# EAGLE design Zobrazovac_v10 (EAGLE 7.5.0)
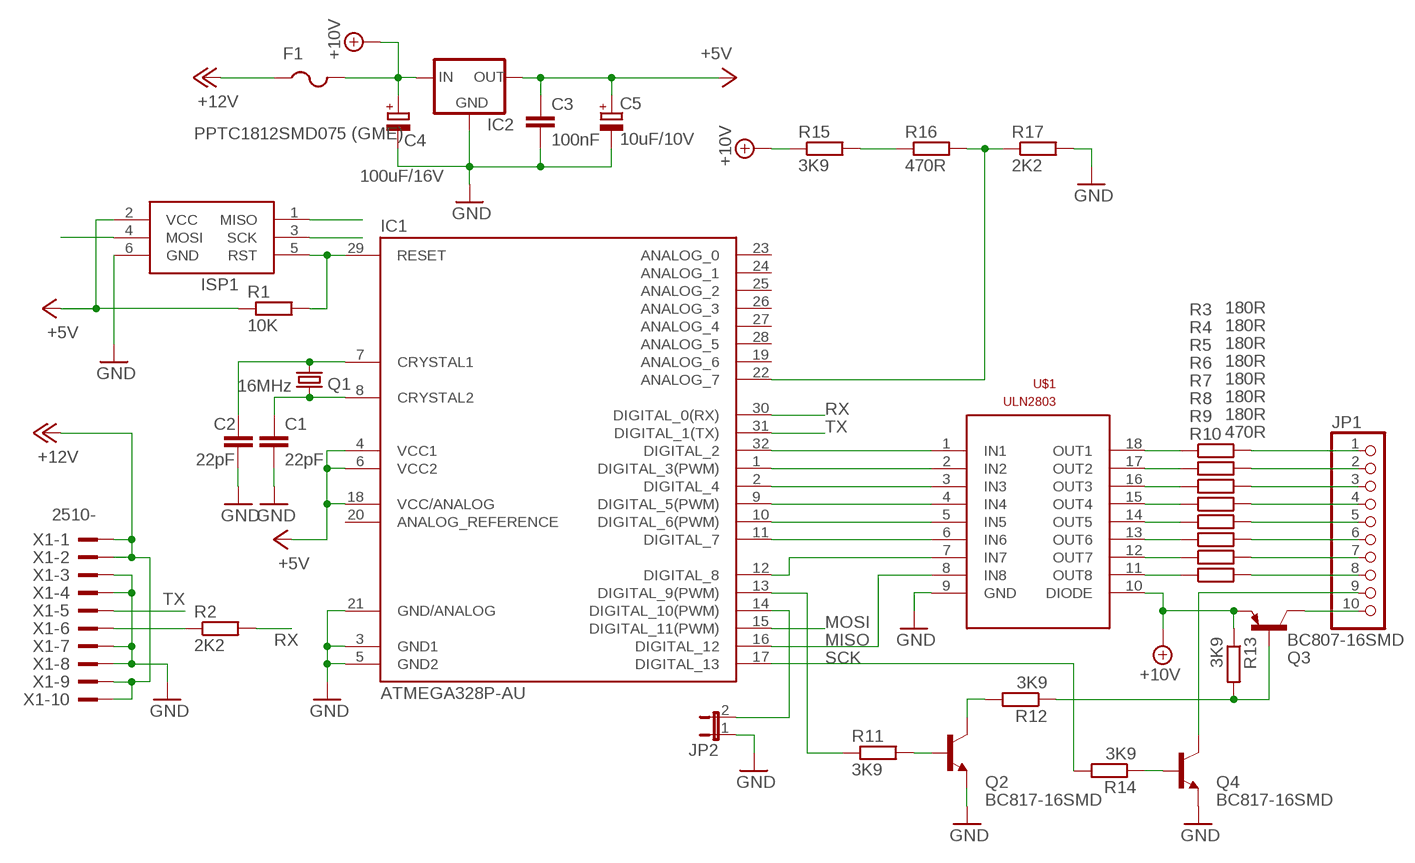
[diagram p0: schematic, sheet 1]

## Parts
C1  22pF  C-EUC1206  [C1206]
C2  22pF  C-EUC1206  [C1206]
C3  100nF  C-EUC1206  [C1206]
C4  100uF/16V  CPOL-EUSMCD  [SMC_D]
C5  10uF/10V  CPOL-EUSMCB  [SMC_B]
F1  PPTC1812SMD075 (GME)  PTCFUSE-1812  [1812]
IC1  ATMEGA328P-AU  ATMEGA168-AU  [TQFP32-08]
IC2  78LXX-SOT89  [SOT89]
ISP1  AVRISP-6  [AVRISP]
JP1  PINHD-1X10  [1X10]
JP2  JP1E  [JP1]
Q1  16MHz  CRYSTALSM49  [SM49]
Q2  BC817-16SMD  [SOT23-BEC]
Q3  BC807-16SMD  [SOT23-BEC]
Q4  BC817-16SMD  [SOT23-BEC]
R1  10K  R-EU_R1206  [R1206]
R2  2K2  R-EU_R1206  [R1206]
R3  180R  R-EU_R1206  [R1206]
R4  180R  R-EU_R1206  [R1206]
R5  180R  R-EU_R1206  [R1206]
R6  180R  R-EU_R1206  [R1206]
R7  180R  R-EU_R1206  [R1206]
R8  180R  R-EU_R1206  [R1206]
R9  180R  R-EU_R1206  [R1206]
R10  470R  R-EU_R1206  [R1206]
R11  3K9  R-EU_R1206  [R1206]
R12  3K9  R-EU_R1206  [R1206]
R13  3K9  R-EU_R1206  [R1206]
R14  3K9  R-EU_R1206  [R1206]
R15  3K9  R-EU_R1206  [R1206]
R16  470R  R-EU_R1206  [R1206]
R17  2K2  R-EU_R1206  [R1206]
U$1  ULN2803  [SO18L]
X1  2510-  [PAK100/2500-10]

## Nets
+5V: C3.1 C5.+ IC1.4(VCC1) IC1.6(VCC2) IC1.18(VCC/ANALOG) IC2.1(OUT) ISP1.2(VCC) R1.1
+10V [10V]: C4.+ F1.2 IC2.3(IN) Q3.E R13.1 R15.1 U$1.10(DIODE)
+12V [10V]: F1.1 X1.1 X1.2 X1.9 X1.10
GND [GND]: C1.2 C2.2 C3.2 C4.- C5.- IC1.3(GND1) IC1.5(GND2) IC1.21(GND/ANALOG) IC2.2(GND) ISP1.6(GND) JP2.1 Q2.E Q4.E R17.2 U$1.9(GND) X1.3 X1.4 X1.7 X1.8
MISO: IC1.16(DIGITAL_12) ISP1.1(MISO) U$1.8(IN8)
MOSI: IC1.15(DIGITAL_11(PWM)) ISP1.4(MOSI)
N$1 [OUT]: R3.1 U$1.18(OUT1)
N$2: R2.1 X1.6
N$3: C2.1 IC1.7(CRYSTAL1) Q1.2
N$4: C1.1 IC1.8(CRYSTAL2) Q1.1
N$5: JP1.1 R3.2
N$6: IC1.32(DIGITAL_2) U$1.1(IN1)
N$7: IC1.1(DIGITAL_3(PWM)) U$1.2(IN2)
N$8: IC1.2(DIGITAL_4) U$1.3(IN3)
N$9: IC1.9(DIGITAL_5(PWM)) U$1.4(IN4)
N$10: IC1.10(DIGITAL_6(PWM)) U$1.5(IN5)
N$11: IC1.11(DIGITAL_7) U$1.6(IN6)
N$12: IC1.12(DIGITAL_8) U$1.7(IN7)
N$13: IC1.14(DIGITAL_10(PWM)) JP2.2
N$14 [OUT]: R4.1 U$1.17(OUT2)
N$15 [OUT]: R5.1 U$1.16(OUT3)
N$16 [OUT]: R6.1 U$1.15(OUT4)
N$17 [OUT]: R7.1 U$1.14(OUT5)
N$18 [OUT]: R8.1 U$1.13(OUT6)
N$19 [OUT]: R9.1 U$1.12(OUT7)
N$20 [OUT]: R10.1 U$1.11(OUT8)
N$21: JP1.2 R4.2
N$22: JP1.3 R5.2
N$23: JP1.4 R6.2
N$24: JP1.5 R7.2
N$25: JP1.6 R8.2
N$26: JP1.7 R9.2
N$27 [10V]: JP1.8 R10.2
N$28: IC1.13(DIGITAL_9(PWM)) R11.1
N$29: Q2.B R11.2
N$30 [10V]: JP1.10 Q3.C
N$31: Q2.C R12.2
N$32: Q3.B R12.1 R13.2
N$33 [10V]: JP1.9 Q4.C
N$34: Q4.B R14.1
N$35: R15.2 R16.1
N$36: IC1.22(ANALOG_7) R16.2 R17.1
RST: IC1.29(RESET) ISP1.5(RST) R1.2
RX: IC1.30(DIGITAL_0(RX)) R2.2
SCK: IC1.17(DIGITAL_13) ISP1.3(SCK) R14.2
TX: IC1.31(DIGITAL_1(TX)) X1.5
Unconnected: IC1.19(ANALOG_6) IC1.20(ANALOG_REFERENCE) IC1.23(ANALOG_0) IC1.24(ANALOG_1) IC1.25(ANALOG_2) IC1.26(ANALOG_3) IC1.27(ANALOG_4) IC1.28(ANALOG_5)

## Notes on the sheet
- RX
- TX
- TX
- MOSI
- RX | MISO
- SCK

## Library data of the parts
C1-C3 = rcl:C-EU: CAPACITOR, European symbol
C4 C5 = rcl:CPOL-EU: POLARIZED CAPACITOR, European symbol
F1 = adafruit:PTCFUSE: PTC fuses, resettable thermistors
IC1 = Arduino-AVR:ATMEGA168
IC2 = v-reg-3:78LXX: VOLTAGE REGULATOR
ISP1 = adafruit:AVRISP: AVR ISP HEADER Standard 6 pin header for AVR programming
JP1 = pinhead:PINHD-1X10: PIN HEADER
JP2 = jumper:JP1E: JUMPER
Q1 = crystal:CRYSTAL: CRYSTAL; OC_FARNELL: unknown; OC_NEWARK: unknown
Q2 Q4 = transistor-npn:BC817*: NPN Transistor
Q3 = transistor-pnp:BC807*: PNP Transistror
R1-R17 = rcl:R-EU_: RESISTOR, European symbol
U$1 = uln2803:ULN2803
X1 = con-3m:2510-: 3M (TM) Pak 100 4-Wall Header Source: 3M; MF: 3M; MPN: 2510-6002UB; OC_FARNELL: 9838244; OC_NEWARK: 46F4725

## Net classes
0 default: width 0.203 mm, drill 0.406 mm, clearance 0.203 mm
1 10V: width 0.61 mm, drill 0.406 mm, clearance 0.203 mm
2 GND: width 0.61 mm, drill 0.406 mm, clearance 0.203 mm
3 OUT: width 0.406 mm, drill 0.406 mm, clearance 0.203 mm

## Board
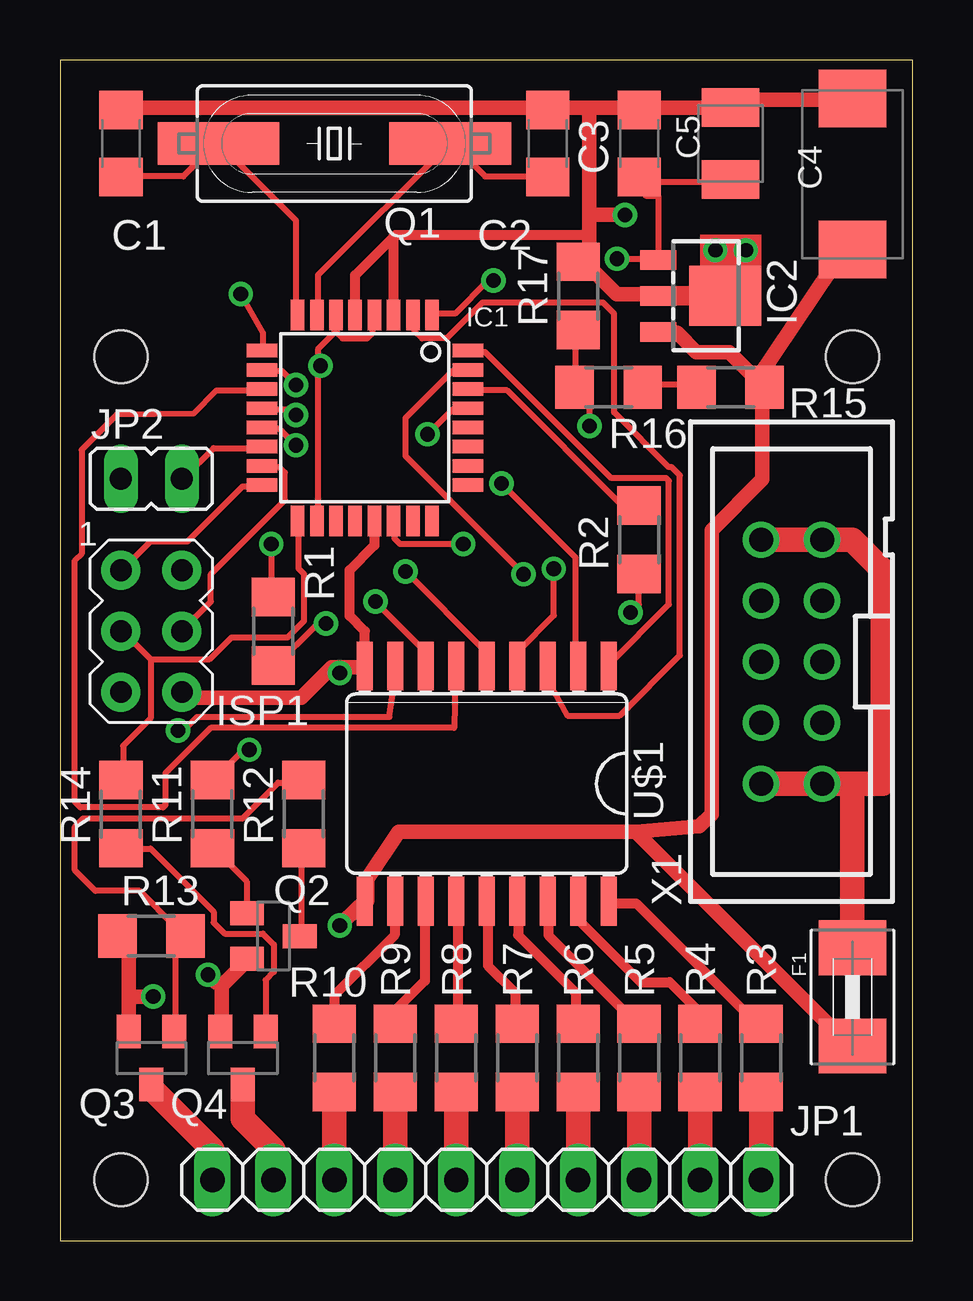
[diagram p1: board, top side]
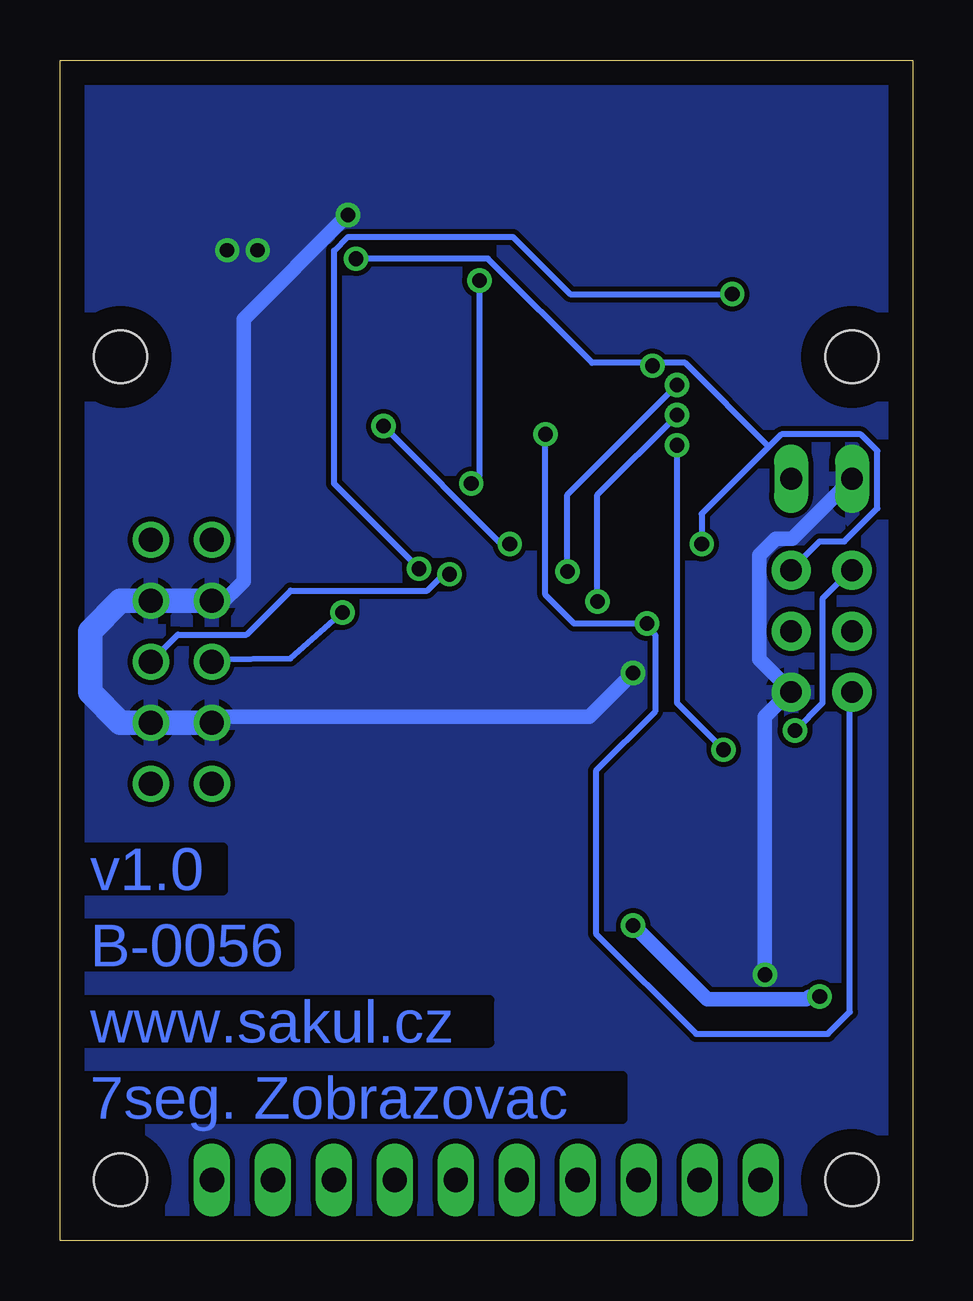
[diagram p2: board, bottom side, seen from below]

Size 35.54 x 49.2 mm. Coordinates in mm from the lower left corner, seen from the top.
Outline: 0,0 35.54,0 35.54,49.2 0,49.2 0,0
Copper layers (1*16): Top 0.035mm / dielectric 1.5mm / Bottom 0.035mm
Design rules "default": minimum track width 10mil, minimum drill 24mil, track to track 8mil, track to pad 8mil, pad to pad 8mil, via to via 8mil, smd to smd 8mil, copper to edge 40mil, drill to drill 8mil, minimum pad ring 10mil, minimum via ring 8mil, stop-mask expansion 4mil, vias tented up to drill 0mil, thermal gap 10mil
Holes 2.2 mm at 2.54,36.83 33.02,36.83 33.02,2.54 2.54,2.54

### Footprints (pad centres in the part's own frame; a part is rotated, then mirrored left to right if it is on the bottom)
C1206 = smd 1.6 x 1.8: 1 -1.4,0; 2 1.4,0
SMC_D = smd 2.4 x 2.8: + -3.15,0; - 3.15,0
SMC_B = smd 1.6 x 2.4: + -1.5,0; - 1.5,0
1812 = smd 2.286 x 2.794: 1 -2.046,0; 2 2.046,0
TQFP32-08 = smd 1.27 x 0.559: 1 -4.293,2.8; 2 -4.293,2; 3 -4.293,1.2; 4 -4.293,0.4; 5 -4.293,-0.4; 6 -4.293,-1.2; 7 -4.293,-2; 8 -4.293,-2.8; 17 4.293,-2.8; 18 4.293,-2; 19 4.293,-1.2; 20 4.293,-0.4; 21 4.293,0.4; 22 4.293,1.2; 23 4.293,2; 24 4.293,2.8 | smd 0.559 x 1.27: 9 -2.8,-4.293; 10 -2,-4.293; 11 -1.2,-4.293; 12 -0.4,-4.293; 13 0.4,-4.293; 14 1.2,-4.293; 15 2,-4.293; 16 2.8,-4.293; 25 2.8,4.293; 26 2,4.293; 27 1.2,4.293; 28 0.4,4.293; 29 -0.4,4.293; 30 -1.2,4.293; 31 -2,4.293; 32 -2.8,4.293
SOT89 = smd 0.8 x 1.5: 1 -1.5,-1.75; 2 0,-1.75; 3 1.5,-1.75 | smd 2.5 x 3: 4 0,1.05
AVRISP = drill 0.9 pad 1.626: 1 -1.27,2.54; 2 1.27,2.54; 3 -1.27,0; 4 1.27,0; 5 -1.27,-2.54; 6 1.27,-2.54
1X10 = drill 1.016 long: 1 -11.43,0; 2 -8.89,0; 3 -6.35,0; 4 -3.81,0; 5 -1.27,0; 6 1.27,0; 7 3.81,0; 8 6.35,0; 9 8.89,0; 10 11.43,0
JP1 = drill 0.914 long: 1 0,-1.27; 2 0,1.27
SM49 = smd 5.08 x 1.778: 1 -4.826,0; 2 4.826,0
SOT23-BEC = smd 1 x 1.4: B -0.95,-1.1; C 0,1.1; E 0.95,-1.1
R1206 = smd 1.6 x 1.803: 1 -1.422,0; 2 1.422,0
SO18L = smd 0.66 x 2.032: 1 -5.08,-4.902; 2 -3.81,-4.902; 3 -2.54,-4.902; 4 -1.27,-4.902; 5 0,-4.902; 6 1.27,-4.902; 7 2.54,-4.902; 8 3.81,-4.902; 9 5.08,-4.902; 10 5.08,4.902; 11 3.81,4.902; 12 2.54,4.902; 13 1.27,4.902; 14 0,4.902; 15 -1.27,4.902; 16 -2.54,4.902; 17 -3.81,4.902; 18 -5.08,4.902
PAK100/2500-10 = drill 1 pad 1.422: 1 -5.08,-1.27; 2 -5.08,1.27; 3 -2.54,-1.27; 4 -2.54,1.27; 5 0,-1.27; 6 0,1.27; 7 2.54,-1.27; 8 2.54,1.27; 9 5.08,-1.27; 10 5.08,1.27

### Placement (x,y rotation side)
C1  2.54,45.72 90 top
C2  20.32,45.72 90 top
C3  24.13,45.72 90 top
C4  33.02,44.45 90 top
C5  27.94,45.72 90 top
F1  33.02,10.16 270 top
IC1  12.7,34.29 270 top
IC2  26.67,39.37 270 top
ISP1  3.81,25.4 0 top
JP1  17.78,2.54 180 top
JP2  3.81,31.75 270 top
Q1  11.43,45.72 0 top
Q2  8.89,12.7 270 top
Q3  3.81,7.62 180 top
Q4  7.62,7.62 180 top
R1  8.89,25.4 270 top
R2  24.13,29.21 90 top
R3  29.21,7.62 270 top
R4  26.67,7.62 270 top
R5  24.13,7.62 270 top
R6  21.59,7.62 270 top
R7  19.05,7.62 270 top
R8  16.51,7.62 270 top
R9  13.97,7.62 270 top
R10  11.43,7.62 270 top
R11  6.35,17.78 270 top
R12  10.16,17.78 270 top
R13  3.81,12.7 0 top
R14  2.54,17.78 90 top
R15  27.94,35.56 180 top
R16  22.86,35.56 180 top
R17  21.59,39.37 90 top
U$1  17.78,19.05 180 top
X1  30.48,24.13 90 top

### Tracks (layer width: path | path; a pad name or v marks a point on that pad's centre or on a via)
+5V  (via drill 0.61)
  Top 0.254: 10.74,36.46 10.74,37.15 11.43,37.83 | 10.74,36.46 10.74,30.06 IC1.18 | 11.43,37.83 11.43,38.52 IC1.6 | IC1.4 13.03,38.52 13.03,37.83 12.8,37.6 11.77,37.6 11.54,37.83 11.43,37.83 | 24.92,43.55 24.92,40.92 IC2.1 24.8,40.92 v23.2,40.92 | 24.92,43.55 24.23,44.23 C3.1 | C5.+ 27.89,44.12 24.97,44.12 24.4,43.55 24.92,43.55 | v8.8,29.03 8.8,26.86 R1.1 | v10.86,36.46 10.74,36.46
  Bottom 0.254: v8.8,29.03 8.8,30.29 6,33.09 | 6,33.09 5.49,33.6 2.17,33.6 1.49,32.92 1.49,30.52 2.86,29.15 3.89,29.15 5.03,28 ISP1.2 | v23.2,40.92 17.72,40.92 13.37,36.58 10.86,36.58 | 10.86,36.58 9.49,36.58 6,33.09 | v10.86,36.46 10.86,36.58
+10V  (via drill 0.61)
  Top 0.61: 29.04,35.88 29.26,35.66 R15.1 29.26,35.32 29.26,31.73 27.15,29.62 27.15,17.78 26.64,17.27 23.99,17.04 | 29.04,35.88 27.89,37.03 26.52,37.03 25.72,37.83 25.03,37.83 IC2.3 | 29.04,35.88 32.92,41.67 32.92,41.26 C4.+ | 2.86,10.17 2.86,12.23 2.4,12.69 R13.1 | 2.86,10.17 2.86,8.8 Q3.E | 23.99,17.04 14.12,17.04 12.8,15.09 12.8,14.17 U$1.10 12.46,13.95 v11.66,13.14 | 23.99,17.04 32.92,8.12 F1.2 | v3.89,10.17 2.86,10.17
  Bottom 0.61: v3.89,10.17 4.33,10.17 4.45,10.06 8.57,10.06 v11.66,13.14
+12V
  Top 1.016: X1.10 X1.9 33.02,29.21 34.29,27.94 34.29,19.05 33.02,19.05 | 33.02,19.05 X1.1 X1.2 | F1.1 33.02,19.05
GND  (via drill 0.6, 0.61)
  Top 0.406: IC1.5 12.3,40.24 13.9,41.84 | 22.06,41.91 13.97,41.91 13.9,41.84 | IC1.3 13.9,41.84 | U$1.9 12.7,25.4 12.06,26.04 12.06,27.94 13.1,28.98 IC1.21
  Top 0.61: IC2.2 24.92,39.43 23.2,39.43 21.95,40.69 21.6,40.69 R17.2 22.06,40.92 22.06,41.91 22.06,42.75 | C1.2 2.63,47.21 20.23,47.21 C2.2 20.57,47.21 22.06,47.21 | 22.06,47.21 24.12,47.21 C3.2 24.35,47.21 27.89,47.21 C5.- 28.12,47.43 28.23,47.55 32.92,47.55 C4.- | 22.06,47.21 22.06,42.75 | 6.74,10.63 6.74,8.8 Q4.E | 6.74,10.63 7.77,11.66 Q2.E | 11.66,23.89 11.32,23.89 10.06,22.63 5.37,22.63 5.14,22.86 ISP1.6 | 11.66,23.89 12.69,23.89 U$1.9 | v6.17,11.09 6.51,10.74 6.74,10.63 | v11.66,23.66 11.66,23.89 | v23.55,42.75 22.06,42.75
  Top 0.813: v27.3,41.27 v28.57,41.27
  Bottom 0.61: v6.17,11.09 6.17,21.83 5.14,22.86 ISP1.6 5.26,23.09 6.4,24.23 6.4,28.57 5.71,29.26 5.03,29.26 JP2.1 | v11.66,23.66 13.49,21.83 28.8,21.83 X1.4 | v23.55,42.75 27.89,38.41 27.89,27.48 28.92,26.45 X1.8
  Bottom 1.016: X1.8 X1.7 33.02,26.67 34.29,25.4 34.29,22.86 33.02,21.59 X1.3 X1.4
  pour Bottom: 0,48.9 35.56,48.9 35.56,0 0,0
MISO  (via drill 0.61)
  Top 0.254: IC1.16 8.34,31.43 7.61,31.43 5.32,29.15 3.77,29.15 2.63,28 ISP1.1 | v4.92,21.26 5.14,21.26 5.71,21.83 13.73,21.83 13.95,23.32 13.95,23.89 U$1.8
  Bottom 0.254: v4.92,21.26 3.77,22.4 3.77,26.75 2.63,27.89 ISP1.1
MOSI
  Top 0.254: IC1.15 8.46,32.23 9.14,32.23 9.37,32 9.37,30.86 6.29,27.77 6.29,26.63 5.14,25.49 ISP1.4
N$1
  Top 0.406: R3.1 29.15,9.14 28.92,9.14 24,14.06 22.86,14.06 U$1.18
N$2  (via drill 0.61)
  Top 0.254: v23.77,26.18 24.12,26.52 24.12,27.77 R2.1
  Bottom 0.254: v23.77,26.18 25.93,24.27 29.15,24.23 X1.6
N$3
  Top 0.254: IC1.7 10.74,38.63 10.74,40.23 16.23,45.72 Q1.2 16.34,45.72 17.72,44.35 20.23,44.35 C2.1
N$4
  Top 0.254: IC1.8 9.83,38.63 9.83,42.52 6.63,45.72 Q1.1 6.51,45.72 5.14,44.35 2.63,44.35 C1.1
N$5
  Top 1.016: R3.2 JP1.1
N$6
  Top 0.254: IC1.32 17.03,37.03 17.72,37.03 22.97,31.77 25.26,31.77 25.38,31.66 25.38,26.52 22.86,24 U$1.1
N$7  (via drill 0.61)
  Top 0.254: v18.06,40.01 17.83,40.01 16.46,38.63 15.54,38.63 IC1.1 | v18.4,31.55 21.49,28.46 21.49,24 U$1.2
  Bottom 0.254: v18.06,40.01 18.06,31.89 v18.4,31.55
N$8
  Top 0.254: IC1.2 14.74,38.52 14.74,37.95 15.09,37.6 16.12,37.6 17.6,39.09 22.63,39.09 23.09,38.63 23.09,34.52 25.38,32.23 25.49,32.23 25.83,31.89 25.83,24.4 23.32,21.88 21.14,21.88 20.34,23.32 20.34,23.89 U$1.3
N$9  (via drill 0.61)
  Top 0.254: v7.53,39.45 8.46,37.83 8.46,37.15 IC1.9 | v20.57,28 20.57,26.06 19.09,24.57 19.09,24 U$1.4
  Bottom 0.254: v7.53,39.45 14.29,39.45 16.68,41.83 23.55,41.83 24.12,41.26 24.12,31.55 v20.57,28
N$10  (via drill 0.61)
  Top 0.254: v9.83,35.66 9.26,36.23 8.46,36.23 IC1.10 | v14.4,27.89 17.72,24.57 17.72,24 U$1.5
  Bottom 0.254: v9.83,35.66 14.4,31.09 v14.4,27.89
N$11
  Top 0.254: IC1.11 8.34,35.43 6.51,35.43 5.56,34.48 2.39,34.44 0.9,32.96 0.9,28.63 0.62,28.35 0.62,18.29 0.85,18.06 4.29,18.06 4.39,18.16 4.39,19.48 6.29,21.37 16.42,21.37 16.46,23.32 16.46,23.89 U$1.6
N$12  (via drill 0.61)
  Top 0.254: v9.83,34.4 9.6,34.63 8.46,34.63 IC1.12 | v13.14,26.63 15.2,24.57 15.2,24 U$1.7
  Bottom 0.254: v9.83,34.4 13.14,31.09 v13.14,26.63
N$13
  Top 0.254: IC1.14 8.34,33.03 6.4,33.03 5.14,31.77 JP2.2
N$14
  Top 0.406: R4.1 26.63,9.14 27.04,9.14 25.4,10.78 24.19,10.78 21.6,13.37 21.6,14.06 U$1.17
N$15
  Top 0.406: R5.1 24.12,9.14 24.12,8.97 20.34,12.74 20.34,14.06 U$1.16
N$16
  Top 0.406: R6.1 21.49,9.14 21.49,10.34 19.09,12.74 19.09,14.06 U$1.15
N$17
  Top 0.406: R7.1 18.97,9.14 18.97,10.32 17.83,11.47 17.83,14.06 U$1.14
N$18
  Top 0.406: R8.1 16.57,9.14 16.57,14.06 U$1.13
N$19
  Top 0.406: R9.1 14.06,9.14 14.06,9.69 15.2,10.83 15.2,14.06 U$1.12
N$20
  Top 0.406: R10.1 11.43,10.22 13.95,12.74 13.95,14.06 U$1.11
N$21
  Top 1.016: R4.2 JP1.2
N$22
  Top 1.016: R5.2 JP1.3
N$23
  Top 1.016: R6.2 JP1.4
N$24
  Top 1.016: JP1.5 R7.2
N$25
  Top 1.016: R8.2 JP1.6
N$26
  Top 1.016: R9.2 JP1.7
N$27
  Top 1.016: R10.2 JP1.8
N$28  (via drill 0.61)
  Top 0.254: v9.83,33.15 9.14,33.83 8.46,33.83 IC1.13 | v7.89,20.46 7.66,20.46 6.4,19.2 R11.1
  Bottom 0.254: v9.83,33.15 9.83,22.4 v7.89,20.46
N$29
  Top 0.254: Q2.B 7.77,13.72 7.77,14.97 6.4,16.34 R11.2
N$30
  Top 1.016: Q3.C 3.81,6.35 6.35,3.81 JP1.10
N$31
  Top 0.254: Q2.C 10.06,12.8 10.06,16.34 R12.2
N$32
  Top 0.254: Q3.B 4.8,8.8 4.8,12.34 5.14,12.69 R13.2 4.8,13.09 3.31,14.58 1.47,14.58 0.62,15.43 0.62,17.26 0.96,17.6 7.61,17.6 9.09,19.09 10.06,19.09 R12.1
N$33
  Top 1.016: Q4.C 7.62,5.08 8.89,3.81 JP1.9
N$34
  Top 0.254: Q4.B 8.57,8.8 8.57,10.86 8.91,11.2 8.91,12.34 8.46,12.8 6.86,12.8 6.4,13.26 6.4,13.72 3.77,16.34 2.63,16.34 R14.1
N$35
  Top 0.254: R16.1 24.35,35.66 26.52,35.66 R15.2
N$36  (via drill 0.61)
  Top 0.254: v16.8,29.03 14.17,29.03 13.95,29.26 13.95,29.95 IC1.22 | v22.06,33.95 22.06,34.98 21.49,35.55 R16.2 21.49,35.66 21.49,37.95 R17.1
  Bottom 0.254: v16.8,29.03 17.14,29.03 v22.06,33.95
N$37
  Top 0.813: 25.4,39.37 26.67,39.37
RST  (via drill 0.61)
  Top 0.254: v15.32,33.6 16.34,34.63 16.92,34.63 IC1.29 | v11.09,25.72 10.74,25.72 8.91,23.89 R1.2
  Bottom 0.254: v15.32,33.6 15.32,26.91 14.12,25.72 v11.09,25.72 11.09,25.6 10.74,25.26 10.74,22.05 13.21,19.58 13.21,12.8 9.03,8.62 3.54,8.62 2.63,9.54 2.63,22.86 ISP1.5
RX
  Top 0.254: IC1.30 17.03,35.43 18.63,35.43 23.43,30.63 24.12,30.63 R2.2
SCK
  Top 0.254: 3.77,24.23 6.24,24.23 7.15,25.15 9.49,25.15 10.17,25.83 10.17,27.77 9.94,28 9.94,29.95 IC1.17 | 3.77,24.23 2.63,25.38 ISP1.3 | 3.77,24.23 3.77,21.77 2.63,20.62 2.63,19.2 R14.2
TX  (via drill 0.61)
  Top 0.254: v19.32,27.77 14.4,32.69 14.4,34.29 16.34,36.23 16.92,36.23 IC1.31
  Bottom 0.254: v19.32,27.77 19.55,27.77 20.23,27.09 25.93,27.09 27.76,25.26 30.63,25.26 31.66,24.23 X1.5
(copper drawn outside any net)
  shapes: Top area x1

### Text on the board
Bottom: v1.0 | B-0056 | www.sakul.cz | 7seg. Zobrazovac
